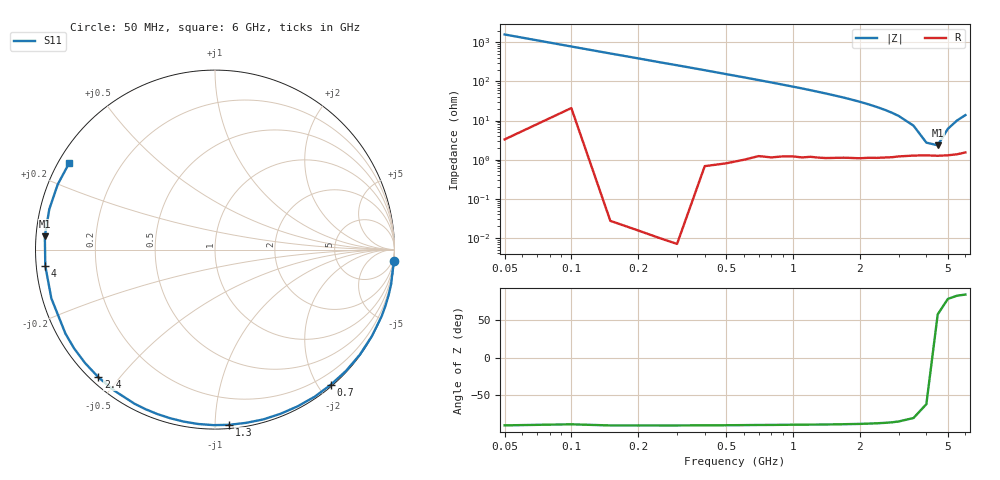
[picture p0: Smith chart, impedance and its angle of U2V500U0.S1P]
! SIEMENS Discrete & RF Semiconductors
! BBY52-02W
! Si Tuning Diode in SCD-80
! VR = 0.5 V
! S-Parameters:  September  1997
# GHz  S  MA  R  50
!  f  S11
! GHz  MAG  ANG
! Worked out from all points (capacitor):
!   34 points, 50 MHz to 6 GHz, reference 50 ohm
!   read as one part to ground: C = 2.03 pF near 50 MHz
!   lowest |Z| = 2.33 ohm at 4.5 GHz (marker M1)
!   series resonance near 4.275 GHz, so ESL is about 680 pH
!   S11 on the Smith chart (normalised r, x): 50 MHz: 0, -32; 700 MHz: 0.02, -2.17; 1.3 GHz: 0.02, -1.09; 2.4 GHz: 0.02, -0.44; 4 GHz: 0.03, -0.05; 6 GHz: 0.03, +0.27
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0.05  0.9999 -3.6
0.15  1 -11.0
0.3  1 -21.8
0.4  0.9983 -28.9
0.5  0.9969 -36.0
0.6  0.9947 -42.8
0.7  0.9914 -49.5
0.8  0.99 -55.9
0.9  0.9871 -62.3
1  0.9849 -68.3
1.1  0.9836 -74.1
1.2  0.9807 -79.8
1.3  0.9795 -85.3
1.4  0.978 -90.5
1.6  0.974 -100.3
1.8  0.9709 -109.3
2  0.9687 -117.6
2.2  0.9654 -125.3
2.4  0.9635 -132.4
2.6  0.9609 -138.9
2.8  0.9588 -145.0
3  0.9557 -150.7
3.5  0.9514 -163.4
4  0.9498 -174.5
4.5  0.951 175.5
5  0.9503 166.3
5.5  0.9485 157.5
6  0.9448 149.3
